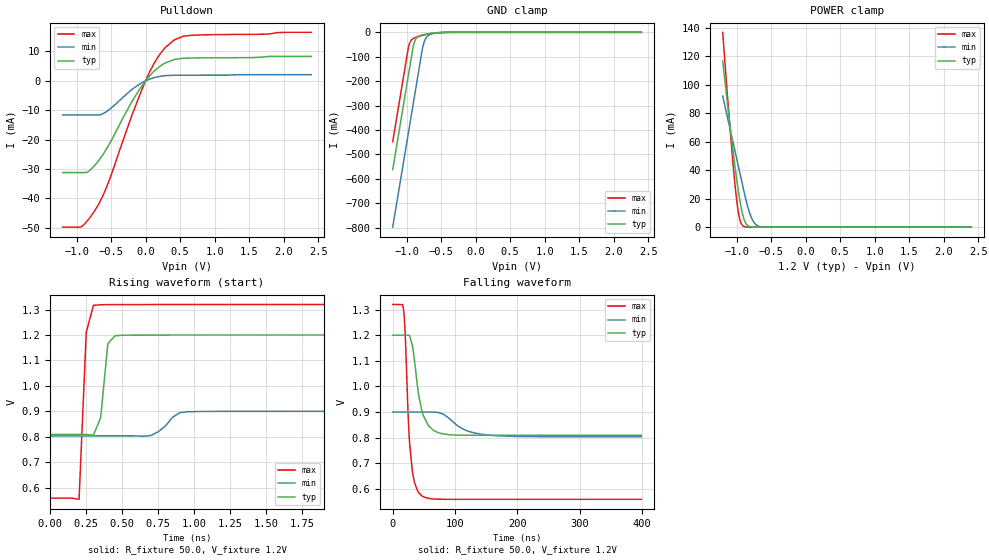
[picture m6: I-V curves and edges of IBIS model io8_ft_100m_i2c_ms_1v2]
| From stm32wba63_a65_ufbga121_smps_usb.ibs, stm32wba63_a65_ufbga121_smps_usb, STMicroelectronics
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[Model]   io8_ft_100m_i2c_ms_1v2
Model_type I/O_open_drain
Polarity   Non-Inverting
Enable   Active-Low
| CAP_THRESHOLD on pad IOFT is "UDTCAPC" :
| Rising=30.0% of vddiom   Falling=70.0% of vddiom
| C_comp min and max val. don't necessarily correlate with the min and max pvt
| but are the smallest and greatest pad capacitance found.
| var   typ   min   max
C_comp   2.85321pF  2.76968pF  2.96421pF
|C_comp_pulldown   2.85321pF  2.76968pF  2.96421pF
Vinl = 450.0mV
Vinh = 660.0mV
Vmeas = 600.0mV   | Reference voltage for timing measurements
Cref  = 50.0pF   | Timing specification test load capacitance value
Rref  = 1.0MOhm   | Timing specification test load resistance value
Vref  = 660.0mV   | Timing specification test load voltage
[Model Spec]
| TIME_THRESHOLD on pin ZII2CV11 is "CMOS" :
| Rising=50.0% of vdd   Falling=50.0% of vdd
Vinl 441.50000mV 335.50000mV 487.50000mV
Vinh 755.50000mV 552.50000mV 839.50000mV
| variable   typ   min   max
[Temperature Range] 25.0 140.0 -40.0
| variable   typ   min   max
[Voltage Range] 1.2V 900.0mV 1.32V
| variable   typ   min   max
[POWER Clamp Reference] 1.2V 900.0mV 1.32V
| variable   typ   min   max
[GND Clamp Reference] 0V 0V 0V
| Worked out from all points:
|   slope of the pulldown table from 0 to 0.18 V, typ, clamps not added: 40.6 ohm
|   GND clamp passes 1 mA (typ) near -0.51 V on its own axis
|   POWER clamp passes 1 mA (typ) near -0.83 V on its own axis
|   rising waveform, R_fixture 50.0, V_fixture 1.2V: 20-80 % time 40.3ps typ, 104ps min, 34.8ps max; typ from 0.809 V to 1.2 V
|   falling waveform, R_fixture 50.0, V_fixture 1.2V: 20-80 % time 15.2ns typ, 36.6ns min, 9.17ns max; typ from 1.2 V to 0.809 V
[POWER Clamp]
-1.2V     116.7mA    92.13mA    136.9mA
-1.09V    69.42mA    68.21mA    67.14mA
-1.02V    41.75mA    52.99mA    28.91mA
-990mV    30.98mA    46.47mA    16.09mA
-970mV    24.36mA    42.12mA    9.575mA
-940mV    15.59mA    35.6mA     3.485mA
-910mV    8.693mA    29.07mA    1.01mA
-860mV    2.259mA    18.59mA    104.6uA
-780mV    143.1uA    6.246mA    2.555uA
-720mV    16.22uA    1.846mA    157.1nA
-650mV    1.267uA    330.3uA    6.118nA
2.4V      0A         0A         0A
[GND Clamp]
-1.2V     -561.6mA   -797.4mA   -447.4mA
-980mV    -187.6mA   -423.4mA   -73.43mA
-960mV    -153.6mA   -389.4mA   -48.26mA
-900mV    -54.17mA   -287.4mA   -24.97mA
-870mV    -29.55mA   -236.4mA   -21.19mA
-830mV    -17.05mA   -168.4mA   -17.42mA
-760mV    -9.921mA   -54.55mA   -11.89mA
-730mV    -8.191mA   -29.78mA   -9.811mA
-690mV    -6.26mA    -14.49mA   -7.318mA
-600mV    -2.976mA   -4.315mA   -3.058mA
-380mV    -57.63uA   -251uA     -19.49uA
2.4V      872.8pA    204.8nA    349.4pA
| variable   typ   min   max
[Pullup Reference] 1.2V 900.0mV 1.32V
| variable   typ   min   max
[Pulldown Reference] 0V 0V 0V
[Pulldown]
-1.2V     -31.2mA    -11.62mA   -49.78mA
-930mV    -31.2mA    -11.62mA   -49.64mA
-830mV    -30.86mA   -11.62mA   -47.25mA
-710mV    -28.04mA   -11.62mA   -43.19mA
-550mV    -22.55mA   -10.2mA    -35.3mA
-200mV    -7.146mA   -2.964mA   -11.89mA
40mV      1.171mA    405.8uA    2.092mA
130mV     3.416mA    1.118mA    6.182mA
230mV     5.302mA    1.613mA    9.763mA
420mV     7.288mA    1.898mA    13.99mA
670mV     7.779mA    1.924mA    15.51mA
2.4V      8.312mA    2.101mA    16.51mA
[Ramp]
dV/dt_r 234.65036mV/727.01809ps 57.87664mV/1.99561ns 456.72484mV/405.08599ps
dV/dt_f 234.6598mV/15.12399ns 57.8955mV/36.14824ns 456.73592mV/8.71481ns
R_load = 50.0
| Removed startup time: 0s 0s 0s  .
| Removed end time: 2.45ns.
[Rising Waveform]
R_fixture   = 50.0
V_fixture   = 1.2V
V_fixture_min = 900.0mV
V_fixture_max = 1.32V
0s        808.9mV    803.5mV    558.8mV
200ps     808.9mV    803.5mV    554mV
250ps     808.9mV    803.5mV    1.211V
300ps     806.3mV    803.5mV    1.317V
350ps     875.2mV    803.5mV    1.319V
400ps     1.166V     803.5mV    1.319V
450ps     1.197V     803.5mV    1.32V
700ps     1.2V       804.9mV    1.32V
950ps     1.2V       898.1mV    1.32V
2.45ns    1.2V       900mV      1.32V
| Removed startup time: 0s 0s 0s  .
| Removed end time: 399.25ns.
[Falling Waveform]
R_fixture   = 50.0
V_fixture   = 1.2V
V_fixture_min = 900.0mV
V_fixture_max = 1.32V
0s        1.2V       900mV      1.32V
17.05ns   1.2V       900mV      1.306V
19.85ns   1.2V       900mV      1.214V
27.15ns   1.198V     900mV      776.7mV
34.95ns   1.103V     900mV      625.4mV
46.6ns    906.8mV    900mV      572.7mV
65.2ns    828.6mV    899.9mV    560.1mV
89.65ns   811.5mV    877.2mV    558.8mV
154.9ns   808.9mV    809.6mV    558.8mV
399.3ns   808.9mV    803.5mV    558.8mV
